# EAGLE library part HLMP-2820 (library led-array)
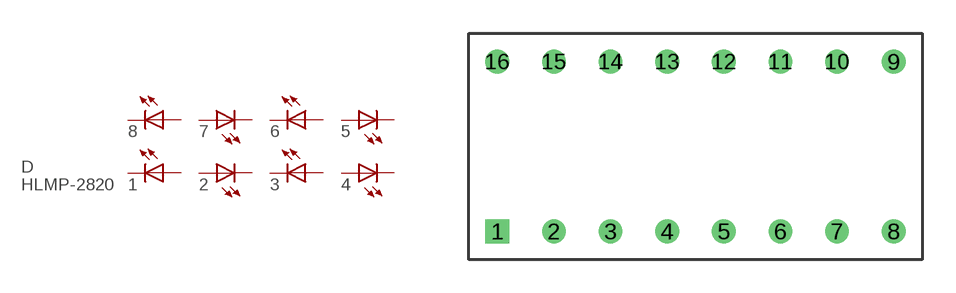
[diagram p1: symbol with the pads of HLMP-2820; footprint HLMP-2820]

Designator prefix D

## HLMP-2820  [HLMP-2820]
1  1  pas
2  2  pas
3  3  pas
4  4  pas
5  5  pas
6  6  pas
7  7  pas
8  8  pas
9  9  pas
10  10  pas
11  11  pas
12  12  pas
13  13  pas
14  14  pas
15  15  pas
16  16  pas

## Footprint HLMP-2820 (pad centres in mm)
drill 0.559 square: 1 1.27,1.27
drill 0.559: 2 3.81,1.27; 3 6.35,1.27; 4 8.89,1.27; 5 11.43,1.27; 6 13.97,1.27; 7 16.51,1.27; 8 19.05,1.27; 9 19.05,8.89; 10 16.51,8.89; 11 13.97,8.89; 12 11.43,8.89; 13 8.89,8.89; 14 6.35,8.89; 15 3.81,8.89; 16 1.27,8.89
